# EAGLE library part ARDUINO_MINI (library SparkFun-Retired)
Arduino Pro Mini footprint
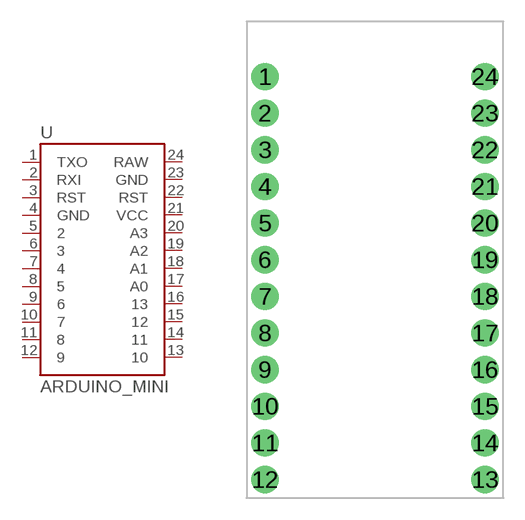
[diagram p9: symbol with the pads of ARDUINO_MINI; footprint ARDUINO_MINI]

Designator prefix -

## ARDUINO_MINI  [ARDUINO_MINI]
1  TXO
2  RXI
3  RST
4  GND
5  2
6  3
7  4
8  5
9  6
10  7
11  8
12  9
13  10
14  11
15  12
16  13
17  A0
18  A1
19  A2
20  A3
21  VCC
22  RST
23  GND
24  RAW

## Footprint ARDUINO_MINI (pad centres in mm)
drill 1.016 pad 1.88: 1 -7.62,12.7; 2 -7.62,10.16; 3 -7.62,7.62; 4 -7.62,5.08; 5 -7.62,2.54; 6 -7.62,0; 7 -7.62,-2.54; 8 -7.62,-5.08; 9 -7.62,-7.62; 10 -7.62,-10.16; 11 -7.62,-12.7; 12 -7.62,-15.24; 13 7.62,-15.24; 14 7.62,-12.7; 15 7.62,-10.16; 16 7.62,-7.62; 17 7.62,-5.08; 18 7.62,-2.54; 19 7.62,0; 20 7.62,2.54; 21 7.62,5.08; 22 7.62,7.62; 23 7.62,10.16; 24 7.62,12.7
